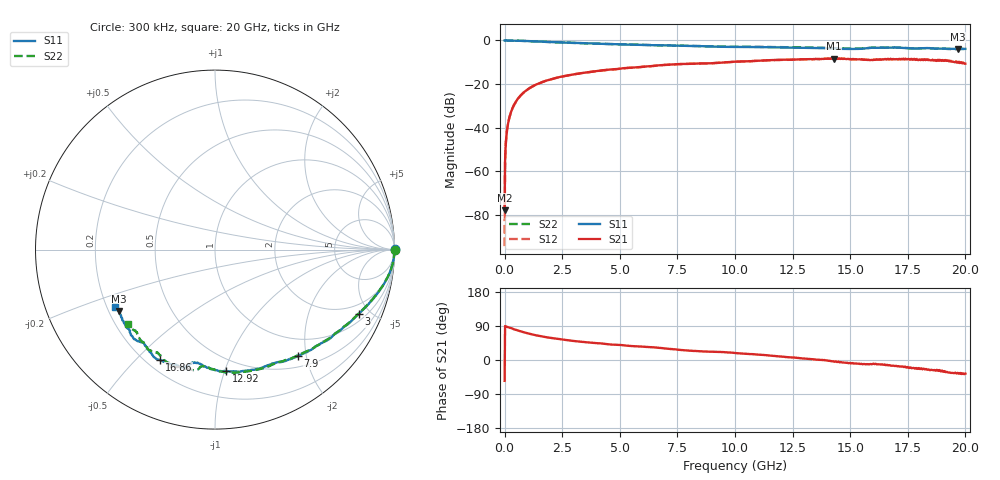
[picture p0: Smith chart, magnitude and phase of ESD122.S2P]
!  2-Port S-parameters saved by WinCal
! VAR MeasName=S-Parameters (CALIBRATED_DATA) read from VNA (N5230A)
! VAR MeasDate=5/30/2017 5:04:31 PM
! VAR NAME=A1_RD
! VAR FILENAME=A1_RD.S2P
! VAR DATE=5/30/2017 5:04:31 PM
! VAR PHYS_PORTS=1,2
! VAR ObjTypeName=DATASET
! VAR IndexType=Frequency
# Hz S MA R 50
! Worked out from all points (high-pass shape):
!   1001 points, 300 kHz to 20 GHz, reference 50 ohm
!   highest |S21| = -8.28 dB at 14.28 GHz (marker M1); lowest = -77.8 dB at 300 kHz (marker M2)
!   |S21| within 3 dB of the highest: 6.814 GHz to end of sweep
!   lowest |S11| = -3.9 dB at 19.66 GHz (marker M3), VSWR 4.49, Z = 12 - j13.9 ohm
!   |S11| at or under -10 dB: nowhere
!   |S22| runs from -4.0 to 0.0 dB; largest |S21 - S12| = 0.018
!   S11 on the Smith chart (normalised r, x): 300 kHz: open; 3 GHz: 1.36, -4.26; 7.9 GHz: 0.67, -1.85; 12.92 GHz: 0.40, -1.01; 16.86 GHz: 0.25, -0.59; 20 GHz: 0.23, -0.25
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300000  1 0.1  0.0001283 -55.0  1.928e-05 -165.1  1 0.0
1.202982e8  0.9993 -1.3  0.009967 87.1  0.009929 87.1  0.9993 -1.3
1.402979e8  0.999 -1.5  0.01157 86.7  0.01154 86.8  0.999 -1.5
2.00297e8  0.9981 -2.2  0.01661 85.4  0.01659 85.4  0.9982 -2.2
2.802958e8  0.9964 -3.1  0.02307 84.1  0.02291 84.2  0.9965 -3.1
5.002925e8  0.9905 -5.3  0.04039 79.3  0.0404 79.2  0.99 -5.4
8.802868e8  0.9747 -9.0  0.06767 72.5  0.06758 72.4  0.9739 -9.1
1.380279e9  0.9495 -13.3  0.09841 65.0  0.09801 65.0  0.9484 -13.3
3.000255e9  0.8778 -24.1  0.1678 50.1  0.1673 50.0  0.8764 -24.0
3.34025e9  0.8659 -26.1  0.1787 48.1  0.1782 48.0  0.8643 -25.9
6.6802e9  0.7764 -44.9  0.269 32.3  0.2666 32.1  0.7782 -44.3
7.900182e9  0.7524 -52.2  0.291 25.4  0.2901 25.4  0.7524 -51.0
1.000015e10  0.7105 -64.2  0.3262 18.6  0.3264 18.4  0.716 -62.1
1.292011e10  0.6802 -84.6  0.3702 4.1  0.3697 4.2  0.6952 -80.6
1.33401e10  0.6769 -88.0  0.3714 2.2  0.3708 2.1  0.6903 -83.8
1.428009e10  0.653 -95.3  0.3856 -3.7  0.3859 -3.9  0.6683 -90.4
1.564007e10  0.6543 -102.5  0.3635 -11.3  0.3626 -11.2  0.6598 -97.3
1.668005e10  0.6868 -114.3  0.3692 -14.1  0.3714 -14.1  0.6847 -107.3
1.686005e10  0.6871 -116.7  0.3714 -14.9  0.3758 -14.5  0.6878 -109.5
1.846002e10  0.6653 -134.9  0.3539 -26.7  0.3651 -26.0  0.6586 -125.4
1.966001e10  0.6358 -147.2  0.3121 -33.9  0.3173 -35.0  0.64 -135.9
2e10  0.6406 -149.9  0.2939 -35.8  0.3029 -37.5  0.6374 -139.5
